FUNCTION_BLOCK FB93
TITLE =Get Enable State
//*****************************************************************************
//* maxon motor ag
//* R&D
//* all rights reserved
//*****************************************************************************
//* Summary:  Read device status
//*
//* Remarks:
//*
//* Created under: STEP7 REV5.2+SP1
//*****************************************************************************
//* History:
//* 19.05.2004 | INA   first release
//*
//*
//*****************************************************************************
//

AUTHOR:INA
FAMILY:StateMac
NAME:GetEnSta
VERSION:00.01


VAR_INPUT

Read : BOOL //A rising edge start the command

  NodeID : BYTE //Adress of the maxon device

END_VAR
VAR_OUTPUT
  Done : BOOL //Data valid flag is TRUE if data were available

  Err : BOOL //Error flag is TRUE if an Error has occured, see ErrNo for more details

  ErrNo : DINT //Contains detailed error information

  IsEnabled : BOOL
END_VAR
VAR
  xEdgeMerker : BOOL //Edge Merker

  xEdgeFlag : BOOL //Edge Flag

  xStep : INT
  xStatusword : WORD
  xOperationEnable : WORD  := W#16#27
END_VAR

BEGIN

NETWORK
TITLE = Activate the service function
//

// SDO Read "Get Enable State"

       U    #Read
       FP   #xEdgeFlag                   // recognize a positiv edge of the Read signal
       =    #xEdgeMerker                 // and set the xEdgeMerker for one cycle to true

       L    #xStep
       L    0
       ==I
       U    #xEdgeMerker
       SPB  nstp                         // iStep = 1 -> fnc1

       L    #xStep                       // jump list
       SPL  List
       SPA  rdef
       SPA  fnc1
       SPA  fncE
List  :SPA  rdef

rdef  :NOP  0
       R    #Done                        // reset Done
       R    #Err                         // reset Error
       L    0
       T    #xStep                       // iStep = 0
       SPA  end

fnc1  :NOP  0
       CALL FC1
         NodeID:=#NodeID
         Index:=DW#16#00006041
         SubIndex:=DW#16#00000000
         RET_VAL:=#Done
         Err:=#Err
         ErrNo:=#ErrNo

       L    DB219.DBW10
       UW   W#16#006F
       T    #xStatusword

       L    #xStatusword
       L    #xOperationEnable
       ==I
       SPB  tdis
       SPA  fdis

tdis  :NOP  0
       S    #IsEnabled                   // set IsEnabled
       SPA  nstp

fdis  :NOP  0
       R    #IsEnabled                   // reset IsEnabled
       SPA  nstp                         // iStep = 1 -> fncE

fncE  :NOP  0
       L    0
       T    #xStep
       SPA  end

nstp  :NOP  0
       L    #xStep
       INC            1
       T    #xStep

end   :NOP  0
END_FUNCTION_BLOCK
